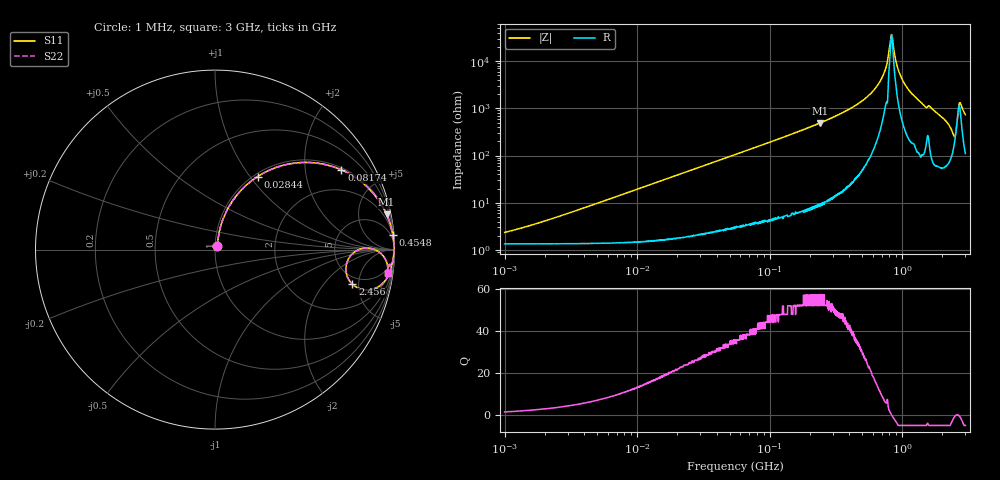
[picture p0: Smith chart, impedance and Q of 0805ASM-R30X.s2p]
!s-Parameter Generated by FASTRON Sdn. Bhd.
!FASTRON P/N : 0805ASM-R30X
!Keysight Technologies: E4991B_MY54100416_A.01.15
!Date: Fri Jun 19 14:52:12 2026
!Version  :Rev00  Fri Jun 19 14:52:12 2026
!Data & Calibration Information:
!Freq  S11  S21  S12  S22
!PortZ  Port1:50+j0  Port2:50+j0
!When reading reference impedance value at option line is always used.
! Remarks : This data is being provided solely for informational purposes.
# Hz S dB R 50
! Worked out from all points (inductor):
!   1601 points, 1 MHz to 3 GHz, reference 50 ohm
!   read as one part in series: L = 308 nH near 2.108 MHz
!   highest Q = 57.1 at 238.5 MHz (marker M1), where L = 323 nH
!   self-resonance near 829.1 MHz
!   S11 on the Smith chart (normalised r, x): 1 MHz: 1.03, +0.04; 28.44 MHz: 1.04, +1.09; 81.74 MHz: 1.08, +3.12; 454.8 MHz: 2, +24; 2.456 GHz: 4.10, -4.17; 3 GHz: 3, -14
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1000000  -32.70 54.0  -0.12 -1.1  -0.12 -1.1  -32.70 54.0
3804036  -22.70 75.3  -0.14 -4.2  -0.14 -4.2  -22.70 75.3
1.447069e7  -11.50 71.4  -0.45 -15.3  -0.45 -15.3  -11.50 71.4
2.843618e7  -6.53 59.7  -1.27 -28.1  -1.27 -28.1  -6.53 59.7
5.504702e7  -2.92 42.8  -3.35 -45.6  -3.35 -45.6  -2.92 42.8
8.173662e7  -1.59 32.2  -5.46 -56.4  -5.46 -56.4  -1.59 32.2
2.083556e8  -0.28 13.4  -12.70 -75.5  -12.70 -75.5  -0.28 13.4
2.384963e8  -0.21 11.6  -13.90 -77.4  -13.90 -77.4  -0.21 11.6
4.548043e8  -0.05 4.7  -21.60 -83.6  -21.60 -83.6  -0.05 4.7
6.719458e8  -0.02 1.6  -30.90 -83.5  -30.90 -83.5  -0.02 1.6
7.42674e8  -0.02 0.9  -36.10 -79.9  -36.10 -79.9  -0.02 0.9
7.925923e8  -0.02 0.3  -43.70 -68.8  -43.70 -68.8  -0.02 0.3
8.167498e8  -0.02 0.1  -48.90 -43.2  -48.90 -43.2  -0.02 0.1
8.416437e8  -0.02 -0.1  -50.20 26.3  -50.20 26.3  -0.02 -0.1
9.538021e8  -0.03 -1.0  -34.90 79.2  -34.90 79.2  -0.03 -1.0
1.153559e9  -0.04 -2.6  -27.00 82.3  -27.00 82.3  -0.04 -2.6
2.092429e9  -0.27 -9.7  -15.40 74.7  -15.40 74.7  -0.27 -9.7
2.347656e9  -0.86 -14.1  -12.00 61.2  -12.00 61.2  -0.86 -14.1
2.455801e9  -2.06 -14.1  -10.40 39.2  -10.40 39.2  -2.06 -14.1
2.594767e9  -1.53 0.6  -15.80 -3.1  -15.80 -3.1  -1.53 0.6
2.727913e9  -0.49 -2.7  -22.90 38.5  -22.90 38.5  -0.49 -2.7
3e9  -0.26 -7.6  -17.50 73.7  -17.50 73.7  -0.26 -7.6
